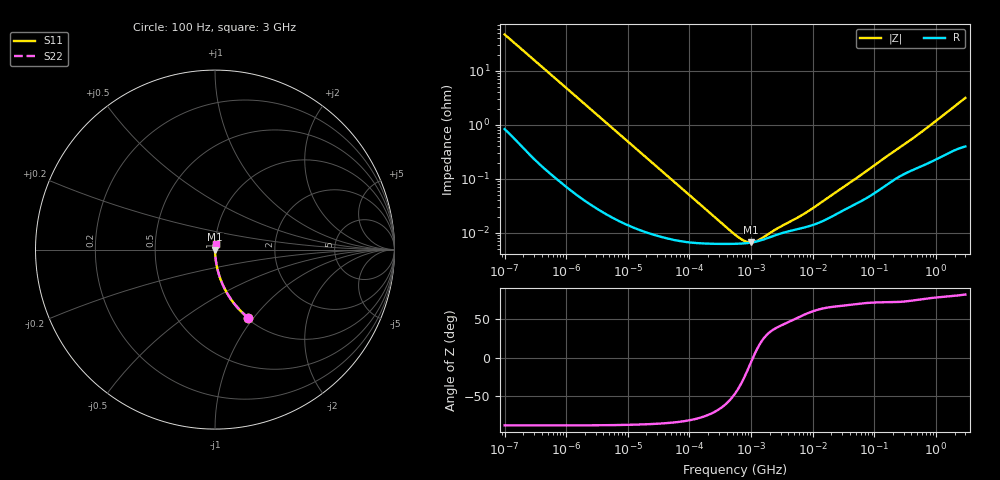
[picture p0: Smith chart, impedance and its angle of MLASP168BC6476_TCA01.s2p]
! MLASP168BC6476_TCA01  S-PARAMETER MODEL  ( Standard Model )
! Model Generated by TAIYO YUDEN Corporation (http://www.ty-top.com)
! Version 1.0
! TAIYO YUDEN Control No. 241206
! Copyright(c) 2024 TAIYO YUDEN CO.,LTD. All Rights Reserved.
! Product Description (link to TY-COMPAS)
! https://ds.yuden.co.jp/TYCOMPAS/or/detail?pn=MLASP168BC6476MTCA01&u=M
! Products Name : Multilayer Ceramic Capacitors
! Characteristics :
!  Capacitance : 47 [uF] , Rated Voltage : 2.5 [V] , TCC : X6S
!  Case Size : 1.6 x 0.8 / 0.063 x 0.031 [mm/inch] , Thickness : 0.8 / 0.031 [mm/inch]
!  (Conditions: Temperature = 25 [degC] , DC Bias Voltage = 0 [V])
! External Node Assignments :
!  1  o---| |---o  2
! GND o---------o GND
! Frequency Range : 100Hz  -  3GHz  [ 401 STEP ]
# MHZ S RI R 50
! Freq[MHz].  S11 Real  S11 Imag  S21 Real  S21 Imag  S12 Real  S12 Imag  S22 Real  S22 Imag
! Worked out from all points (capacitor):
!   401 points, 100 Hz to 3 GHz, reference 50 ohm
!   read as one part in series: C = 33.7 uF near 109 Hz
!   lowest |Z| = 6.68 mohm at 1.001 MHz (marker M1)
!   series resonance near 1.075 MHz, so ESL is about 650 pH
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0.0001  0.1857 -0.3801  0.8143 0.3801  0.8143 0.3801  0.1857 -0.3801
0.000114  0.1509 -0.3493  0.8491 0.3493  0.8491 0.3493  0.1509 -0.3493
0.000147  0.0975 -0.2883  0.9025 0.2883  0.9025 0.2883  0.0975 -0.2883
0.000183  0.0666 -0.2413  0.9334 0.2413  0.9334 0.2413  0.0666 -0.2413
0.000269  0.0327 -0.1706  0.9673 0.1706  0.9673 0.1706  0.0327 -0.1706
0.000396  0.016 -0.1183  0.984 0.1183  0.984 0.1183  0.016 -0.1183
0.000789  0.00456 -0.0605  0.9954 0.0605  0.9954 0.0605  0.00456 -0.0605
0.001788  0.00116 -0.027  0.9988 0.027  0.9988 0.027  0.00116 -0.027
0.005476  0.000274 -0.00891  0.9997 0.00891  0.9997 0.00891  0.000274 -0.00891
0.031977  8.93e-05 -0.00155  0.9999 0.00155  0.9999 0.00155  8.93e-05 -0.00155
0.461094  6.28e-05 -8.98e-05  0.9999 8.98e-05  0.9999 8.98e-05  6.28e-05 -8.98e-05
0.547723  6.3e-05 -6.86e-05  0.9999 6.86e-05  0.9999 6.86e-05  6.3e-05 -6.86e-05
1.000599  6.65e-05 -6.65e-06  0.9999 6.65e-06  0.9999 6.65e-06  6.65e-05 -6.65e-06
1.827928  8.01e-05 4.7e-05  0.9999 -4.7e-05  0.9999 -4.7e-05  8.01e-05 4.7e-05
2.079876  8.45e-05 5.76e-05  0.9999 -5.76e-05  0.9999 -5.76e-05  8.45e-05 5.76e-05
5.843389  0.000119 0.000156  0.9999 -0.000156  0.9999 -0.000156  0.000119 0.000156
9.794414  0.000139 0.000245  0.9999 -0.000245  0.9999 -0.000245  0.000139 0.000245
52.48047  0.000355 0.000991  0.9996 -0.000991  0.9996 -0.000991  0.000355 0.000991
175.1444  0.000849 0.00269  0.9992 -0.00269  0.9992 -0.00269  0.000849 0.00269
513.708  0.00165 0.00643  0.9983 -0.00643  0.9983 -0.00643  0.00165 0.00643
2752.553  0.00469 0.0288  0.9953 -0.0288  0.9953 -0.0288  0.00469 0.0288
3000  0.00495 0.0312  0.9951 -0.0312  0.9951 -0.0312  0.00495 0.0312
